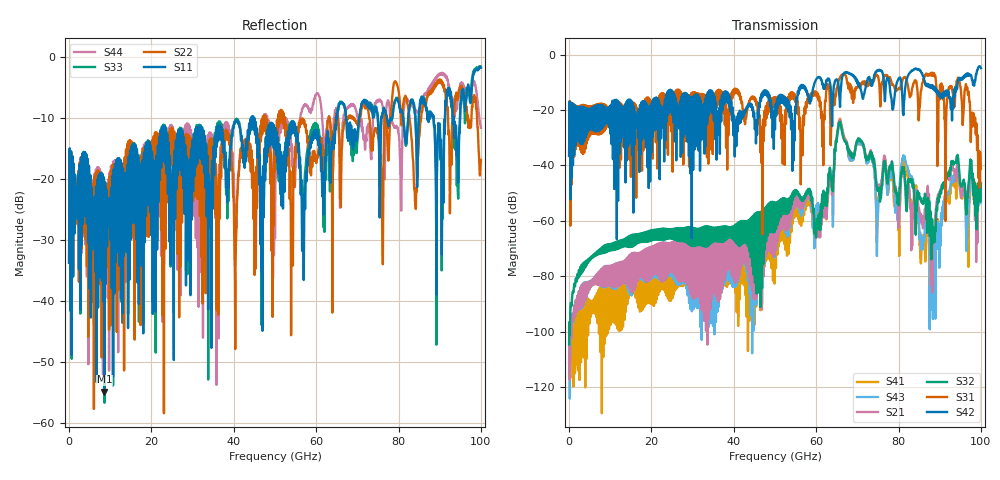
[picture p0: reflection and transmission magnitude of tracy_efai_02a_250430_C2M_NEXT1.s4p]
!! PART DESCRIPTION: TE 224G+ VSR Channel- Chip to module, IO connector to CPC(Co-packaged connector) through over the board cable
!! CHANNEL DESCRIPTION: Module trace -> Mated IO 224G+ Connector -> Internal Cable Termination -> 30AWG 300mm Cable -> Cable
!!  termination + CPC connector(No footprint or package included)
!! MODEL REVISION:  Rev 3, Created on April 29, 2025
!! MODEL STATUS: Development
!! MODEL GEOMETRY: NEXT1
!! MODEL FREQUENCY RANGE: 0 GHz to 100 GHz in 10.00 MHz frequency steps
!! PORT DEFINITIONS:
!! Port  1  ----->  Module Side  -->  Module Side  <-----  Port  2
!! Port  3  ----->  Module Side  -->  Module Side  <-----  Port  4
# HZ S MA R 45.000000
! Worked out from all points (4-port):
!   10000 points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, 10 MHz to 100 GHz, reference 45 ohm
!   strongest paths, dB at 10 MHz, 25.01 GHz, 50.01 GHz, 75.01 GHz, 100 GHz:
!     S42: -36.5, -18.7, -26.9, -5.6, -4.8
!     S31: -36.5, -17.8, -16.0, -7.7, -40.6
!     S32: -104.7, -64.9, -55.4, -48.8, -46.6
!     S21: -111.3, -75.0, -58.4, -48.0, -48.0
!     S43: -111.3, -74.8, -59.1, -57.4, -51.4
!     S41: -116.4, -81.2, -63.0, -54.1, -46.4
!   lowest |S11| = -54.9 dB at 8.6 GHz (marker M1), VSWR 1.00, Z = 44.9 + j0.15 ohm
!   |S11| at or under -10 dB: start of sweep to 44.32 GHz; 44.72 GHz to 64.9 GHz (20.18 GHz wide, 36.8 % of centre); 67.23 GHz to 70.41 GHz (3.185 GHz wide, 4.63 % of centre)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
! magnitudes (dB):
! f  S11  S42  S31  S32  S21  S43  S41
! 10 MHz  -33.8  -36.5  -36.5  -104.7  -111.3  -111.3  -116.4
! 8.6 GHz  -54.9  -21.7  -27.5  -70.2  -80.4  -80.3  -89.8
! 60.27 GHz  -13.4  -8.4  -15.4  -60.5  -62.9  -56.3  -57.9
! 65.77 GHz  -7.6  -18.2  -8.3  -24.2  -23.5  -23.8  -23.1
! 88.56 GHz  -10.8  -11.9  -6.8  -62.5  -65.4  -66.8  -70.6
! 94.06 GHz  -14.0  -12.1  -9.9  -37.8  -43.5  -41.8  -48.4
! 100 GHz  -1.8  -4.8  -40.6  -46.6  -48.0  -51.4  -46.4
